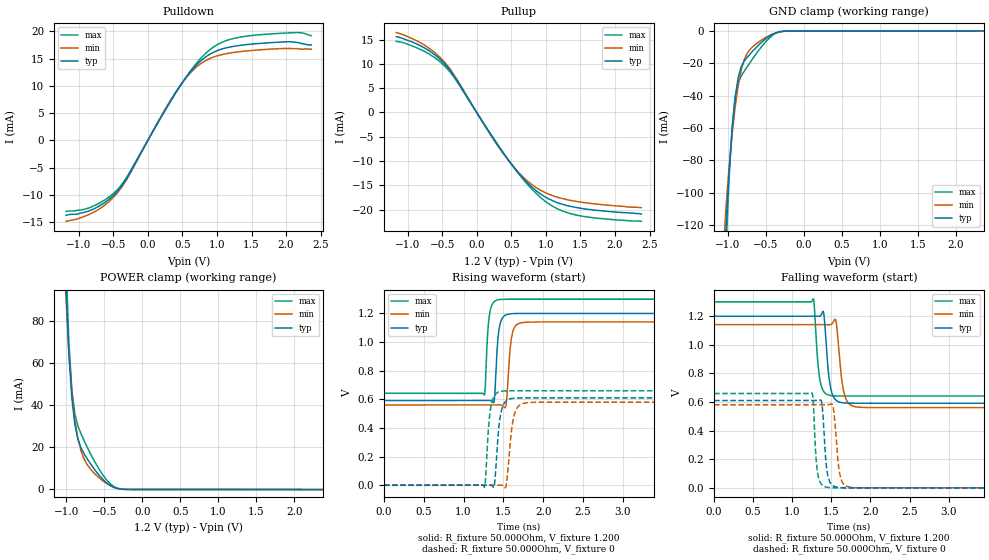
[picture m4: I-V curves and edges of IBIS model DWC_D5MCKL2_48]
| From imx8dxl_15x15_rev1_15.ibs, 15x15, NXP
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[Model] DWC_D5MCKL2_48
Model_type   I/O
Polarity   Non-Inverting
Enable   Active-High
C_comp   1.264pF   1.181pF   1.367pF
C_comp_pullup   285.781fF   264.560fF   312.242fF
C_comp_pulldown 969.546fF   903.205fF   1.049pF
Vinh = 820.000mV
Vinl = 380.000mV
Vmeas = 600.000mV
Vref = 600.000mV
Rref = 50Ohms
Cref = 5pF
[Model Spec]
Vinh   820.000mV   790.000mV   870.000mV
Vinl   380.000mV   350.000mV   430.000mV
Vmeas   600.000mV   570.000mV   650.000mV
Vref   600.000mV   570.000mV   650.000mV
D_overshoot_ampl_h 0.35 NA   NA
D_overshoot_ampl_l 0.35 NA   NA
D_overshoot_area_l 150.000p NA   NA
D_overshoot_area_h 150.000p NA   NA
[Receiver Thresholds]
Vcross_low = 480.000mV
Vcross_high = 720.000mV
Vdiff_ac = 440.000mV
Vdiff_dc = 260.000mV
Tdiffslew_ac = 10.000ns
[Temperature Range]   25.000   125.000   -40.000
[Voltage Range]   1.200V   1.140V   1.300V
[GND Clamp Reference]   0.00V   0.00V   0.00V
[C Comp Corner]
| variable   typ   min   max
C_comp 1.264pF   1.367pF   1.181pF
C_comp_pullup 285.781fF   312.242fF   264.560fF
C_comp_pulldown 969.546fF   1.049pF   903.205fF
[Pulldown Reference]   0.00V   0.00V   0.00V
[POWER Clamp Reference]   1.200V   1.140V   1.300V
[Pullup Reference]   1.200V   1.140V   1.300V
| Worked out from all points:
|   slope of the pulldown table from 0 to 0.18 V, typ, clamps not added: 44.5 ohm
|   slope of the pullup table from 0 to 0.18 V, typ, clamps not added: 44.6 ohm
|   GND clamp passes 1 mA (typ) near -0.36 V on its own axis
|   POWER clamp passes 1 mA (typ) near -0.38 V on its own axis
|   rising waveform, R_fixture 50.000Ohm, V_fixture 1.200: 20-80 % time 43ps typ, 49ps min, 40.6ps max; typ from 0.591 V to 1.2 V
|   rising waveform, R_fixture 50.000Ohm, V_fixture 0: 20-80 % time 57.4ps typ, 66.7ps min, 51.8ps max; typ from 0 V to 0.609 V
|   falling waveform, R_fixture 50.000Ohm, V_fixture 1.200: 20-80 % time 61.5ps typ, 70.4ps min, 55.5ps max; typ from 1.2 V to 0.591 V
|   falling waveform, R_fixture 50.000Ohm, V_fixture 0: 20-80 % time 48.4ps typ, 57ps min, 42.4ps max; typ from 0.609 V to 0 V
[GND Clamp]
-1.182V   -339.3mA   -254.8mA   -426.6mA
-1.064V   -163.5mA   -137.8mA   -190.4mA
-1.024V   -121.1mA   -108.6mA   -134.3mA
-984.8mV  -87.5mA    -84.22mA   -91.46mA
-945.5mV  -61.36mA   -64.12mA   -60.5mA
-906.1mV  -41.91mA   -47.62mA   -41.1mA
-866.7mV  -29.17mA   -34.43mA   -32.17mA
-827.3mV  -22.35mA   -24.56mA   -28.07mA
-748.5mV  -16.34mA   -13.87mA   -22.22mA
-590.9mV  -8.454mA   -6.602mA   -11.71mA
-275.8mV  -116.4uA   -248.8uA   -84.78uA
2.364V    136.6uA    111.3uA    170.2uA
[Power Clamp]
-1.164V   362.5mA    268.1mA    465.2mA
-1.006V   98.99mA    92.43mA    111.8mA
-966.7mV  64.74mA    65.63mA    70.25mA
-927.3mV  43.55mA    46.45mA    47.41mA
-887.9mV  31.08mA    33.31mA    36.05mA
-848.5mV  24.04mA    24.48mA    30.35mA
-809.1mV  19.97mA    18.62mA    26.67mA
-690.9mV  12.66mA    10.09mA    17.63mA
-493.9mV  3.911mA    3.404mA    5.643mA
-375.8mV  976.4uA    1.116mA    1.399mA
-257.6mV  56.8uA     160.4uA    65.6uA
2.382V    -68.29uA   -58.74uA   -77.9uA
[Pulldown]
-1.182V   -13.7mA    -14.8mA    -13mA
-787.9mV  -12.57mA   -13.18mA   -12.01mA
-590.9mV  -11.07mA   -11.52mA   -10.62mA
-433.3mV  -9.208mA   -9.488mA   -8.909mA
-275.8mV  -6.289mA   -6.51mA    -6.115mA
354.5mV   7.765mA    7.888mA    7.678mA
551.5mV   11.5mA     11.44mA    11.54mA
748.5mV   14.38mA    13.9mA     14.79mA
984.8mV   16.34mA    15.41mA    17.39mA
1.261V    17.27mA    16.14mA    18.73mA
2.127V    18mA       16.8mA     19.74mA
2.364V    17.5mA     16.7mA     19.2mA
[Pullup]
-1.164V   15.6mA     16.45mA    14.65mA
-730.3mV  13.08mA    13.63mA    12.38mA
-572.7mV  11.5mA     11.91mA    10.92mA
-415.1mV  9.21mA     9.482mA    8.825mA
-297mV    6.851mA    7.079mA    6.615mA
372.7mV   -8.112mA   -8.2mA     -8.037mA
609.1mV   -12.53mA   -12.38mA   -12.63mA
806.1mV   -15.45mA   -14.92mA   -15.9mA
1.042V    -17.79mA   -16.82mA   -18.8mA
1.318V    -19.2mA    -17.98mA   -20.66mA
1.712V    -20.11mA   -18.82mA   -21.71mA
2.382V    -20.9mA    -19.6mA    -22.4mA
[Ramp]
R_load=50.000Ohm
dV/dt_r   365.130mV/50.500ps  347.458mV/58.000ps  394.470mV/46.000ps
dV/dt_f   365.130mV/56.000ps  347.458mV/64.500ps  394.470mV/49.500ps
[Rising waveform]
R_fixture=50.000Ohm
V_fixture=1.200
V_fixture_min=1.140
V_fixture_max=1.300
0s        590.7mV    560.1mV    641.5mV
1.263ns   590.7mV    560.1mV    629.6mV
1.323ns   591.4mV    560.1mV    1.179V
1.383ns   579.5mV    560mV      1.279V
1.423ns   961.7mV    560.5mV    1.291V
1.464ns   1.135V     560.4mV    1.296V
1.534ns   1.188V     558.2mV    1.297V
1.614ns   1.197V     1.061V     1.298V
1.744ns   1.198V     1.135V     1.298V
10ns      1.198V     1.139V     1.298V
[Rising waveform]
R_fixture=50.000Ohm
V_fixture=0
0s        204.3nV    5.107uV    28.05nV
1.263ns   -2.733uV   3.889uV    -13.86mV
1.343ns   1.201mV    8.612uV    548mV
1.383ns   -14.02mV   -88.27uV   622mV
1.444ns   407.7mV    870.7uV    651.3mV
1.484ns   537.9mV    171.1uV    656.2mV
1.534ns   587.8mV    -7.39mV    658.3mV
1.644ns   607.4mV    503.6mV    659mV
1.794ns   609.5mV    575.4mV    659.1mV
10ns      609.4mV    579.5mV    658.6mV
[Falling waveform]
R_fixture=50.000Ohm
V_fixture=1.200
V_fixture_min=1.140
V_fixture_max=1.300
0s        1.198V     1.139V     1.298V
1.273ns   1.198V     1.139V     1.317V
1.353ns   1.198V     1.139V     755mV
1.403ns   1.217V     1.139V     671.2mV
1.464ns   795.2mV    1.138V     647.5mV
1.504ns   666.9mV    1.144V     643.3mV
1.564ns   609.4mV    1.148V     641.4mV
1.674ns   592.3mV    638.3mV    640.8mV
1.834ns   590.4mV    563.9mV    640.8mV
10ns      590.6mV    560.1mV    641.3mV
[Falling waveform]
R_fixture=50.000Ohm
V_fixture=0
0s        609.3mV    579.5mV    658.4mV
1.253ns   609.3mV    579.5mV    662.1mV
1.323ns   609mV      579.5mV    108.5mV
1.383ns   569.1mV    579.5mV    18.65mV
1.454ns   86.46mV    579.5mV    2.963mV
1.524ns   13.63mV    561mV      522.1uV
1.584ns   3.7mV      190.9mV    121.6uV
1.624ns   1.644mV    60.17mV    48.4uV
1.754ns   128.2uV    3.942mV    8.325uV
10ns      586.3nV    5.419uV    311.2nV
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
